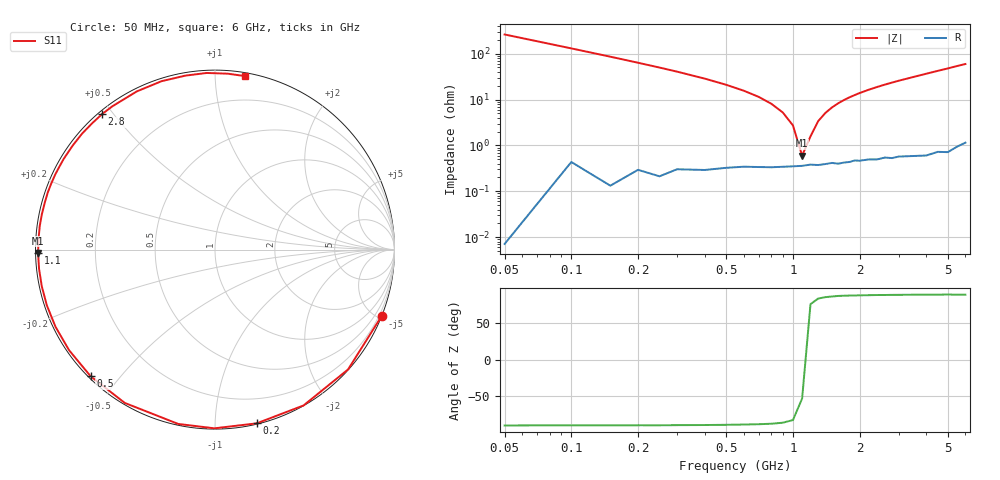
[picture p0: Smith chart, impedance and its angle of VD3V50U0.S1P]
! Infineon Technologies  Discrete & RF Semiconductors
! BBY 55-03
! Si Tuning Diode in SOD323
! VR = 3.5 V
! S-Parameters:  June  1999
# GHz  S  MA  R  50
!  f  S11
! GHz  MAG  ANG
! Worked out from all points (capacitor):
!   34 points, 50 MHz to 6 GHz, reference 50 ohm
!   read as one part to ground: C = 12.1 pF near 50 MHz
!   lowest |Z| = 599 mohm at 1.1 GHz (marker M1)
!   series resonance near 1.124 GHz, so ESL is about 1.7 nH
!   S11 on the Smith chart (normalised r, x): 50 MHz: 0.00, -5.24; 200 MHz: 0.01, -1.27; 500 MHz: 0.01, -0.42; 1.1 GHz: 0.01, -0.01; 2.8 GHz: 0.01, +0.47; 6 GHz: 0.02, +1.19
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0.05  1 -21.6
0.1  0.9978 -42.0
0.15  0.9987 -60.4
0.2  0.9955 -76.5
0.25  0.9958 -90.2
0.3  0.9927 -101.9
0.4  0.9912 -120.5
0.5  0.989 -134.5
0.6  0.9876 -145.4
0.7  0.9872 -154.2
0.8  0.987 -161.7
0.9  0.9866 -168.1
1  0.9861 -173.8
1.1  0.9858 -178.9
1.3  0.9852 172.3
1.6  0.9846 161.2
1.8  0.9835 154.8
2  0.9829 149.0
2.2  0.9823 143.7
2.4  0.9828 138.8
2.8  0.9828 129.8
3  0.9821 125.6
3.5  0.9832 116.3
4  0.9844 107.6
4.5  0.9832 99.7
5  0.9852 92.7
5.5  0.9827 85.9
6  0.9812 80.1
